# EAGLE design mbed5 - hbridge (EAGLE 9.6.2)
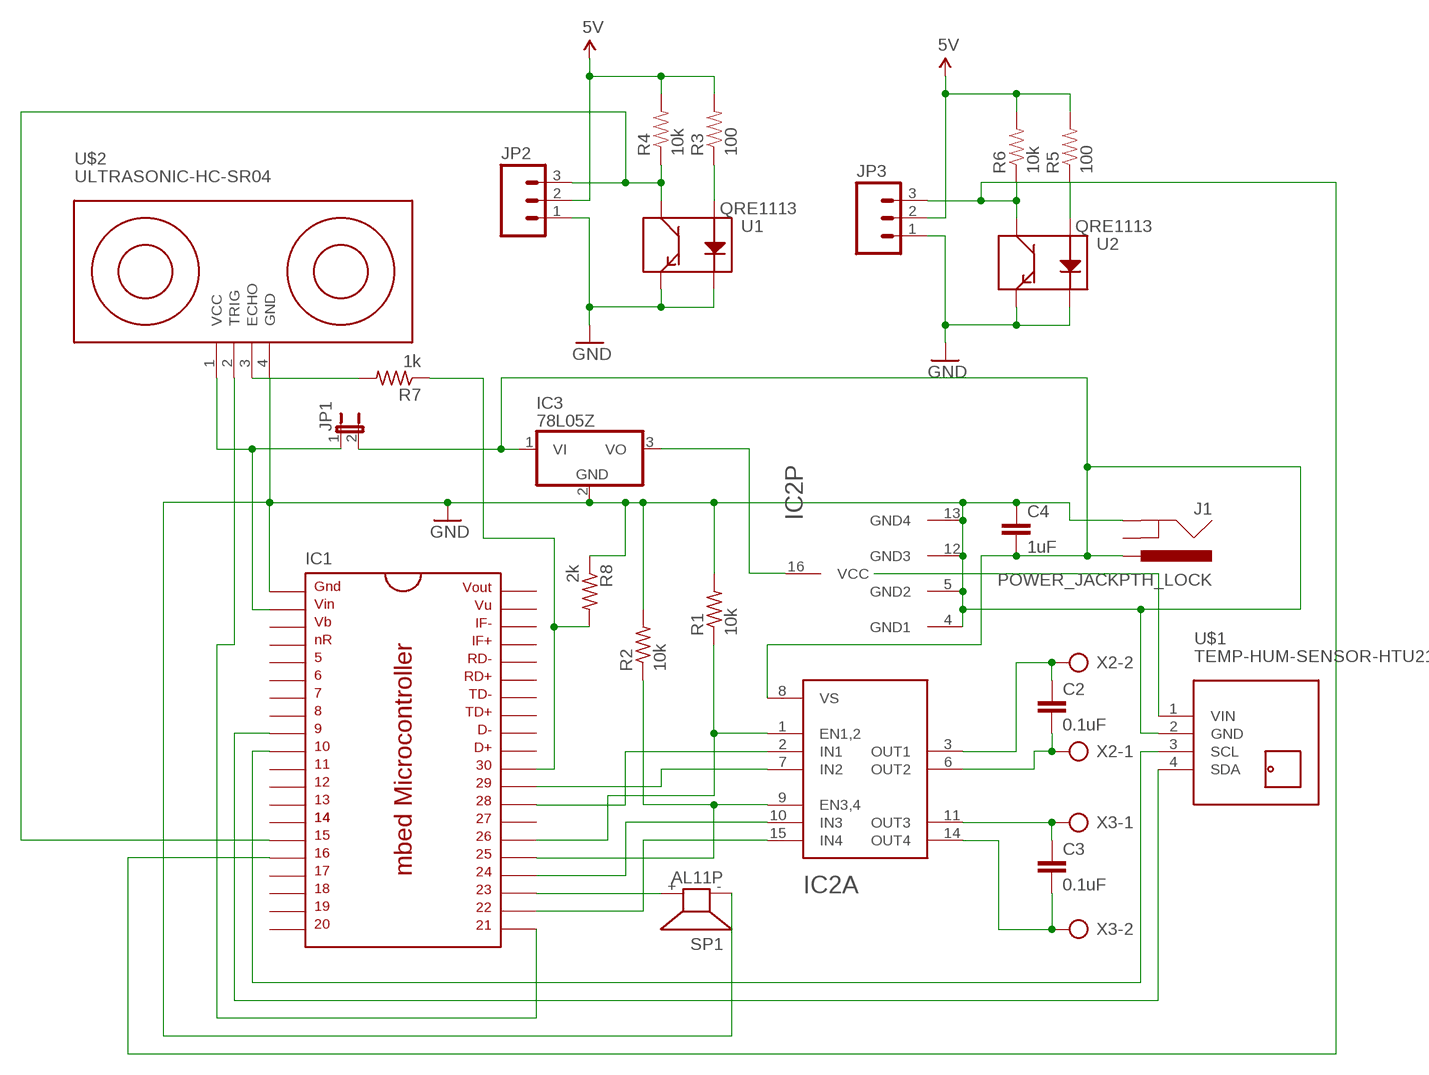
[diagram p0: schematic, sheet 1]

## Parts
C2  0.1uF  C5/3.5  [C5B3.5]
C3  0.1uF  C5/3.5  [C5B3.5]
C4  1uF  C5/3.5  [C5B3.5]
IC1  MBED_MICROCONTROLLER  [DIL40_0.9]
IC2  L293D  [DIP16]
IC3  78L05Z  [TO92]
J1  POWER_JACKPTH_LOCK  [POWER_JACK_PTH_LOCK]
JP1  JUMPER-2PTH  [1X02]
JP2  M03SMD_RA_MALE  [1X03_SMD_RA_MALE]
JP3  M03SMD_RA_MALE  [1X03_SMD_RA_MALE]
R1  10k  R-US_0207/10  [0207/10]
R2  10k  R-US_0207/10  [0207/10]
R3  100  100-1%  [0402-RES]
R4  10k  10KOHM1/10W1%(0603)  [0402-RES]
R5  100  100-1%  [0402-RES]
R6  10k  10KOHM1/10W1%(0603)  [0402-RES]
R7  1k  R-US_0207/10  [0207/10]
R8  2k  R-US_0207/10  [0207/10]
SP1  AL11P  [AL11P]
U1  QRE1113  [QRE1113]
U2  QRE1113  [QRE1113]
U$1  TEMP-HUM-SENSOR-HTU21D  [TEMP-HUM-SENSOR-HTU21D]
U$2  ULTRASONIC-HC-SR04  [ULTRASONIC-HC-SR04]
X2  AK300/2  [AK300/2]
X3  AK300/2  [AK300/2]

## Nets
5V: JP2.2 JP3.2 R3.2 R4.2 R5.2 R6.2
GND: JP2.1 JP3.1 U1.2(K) U1.4(E) U2.2(K) U2.4(E)
N$1: IC1.22 IC2.15(A:IN4)
N$2: IC1.24 IC2.10(A:IN3)
N$3: IC1.25 IC2.9(A:EN3,4) R2.1
N$4: IC1.28 IC2.2(A:IN1)
N$5: IC1.29 IC2.7(A:IN2)
N$6: IC1.26 IC2.1(A:EN1,2) R1.1
N$7: IC1.9 U$1.4(SDA)
N$8: C2.1 IC2.3(A:OUT1) X2.2
N$9: C2.2 IC2.6(A:OUT2) X2.1
N$10: C3.1 IC2.11(A:OUT3) X3.1
N$11: C3.2 IC2.14(A:OUT4) X3.2
N$12: IC2.16(P:VCC) IC3.3(VO)
N$13: IC1.2 JP1.1 U$2.1(VCC)
N$14: C4.1 C4.2 IC1.1 IC2.4(P:GND1) IC2.5(P:GND2) IC2.8(A:VS) IC2.12(P:GND3) IC2.13(P:GND4) IC3.1(VI) IC3.2(GND) J1.GND J1.PWR JP1.2 R1.2 R2.2 R8.1 SP1.- U$1.2(GND) U$2.4(GND) ; supply symbol labelled GND
N$15: IC1.10 U$1.3(SCL)
N$16: IC1.23 SP1.+
N$17: U$1.1(VIN)
N$18: IC1.21 U$2.2(TRIG)
N$20: R3.1 U1.1(A)
N$21: IC1.15 JP2.3 R4.1 U1.3(C)
N$22: R7.2 U$2.3(ECHO)
N$23: R5.1 U2.1(A)
N$24: IC1.16 JP3.3 R6.1 U2.3(C)
N$25: IC1.30 R7.1 R8.2
Unconnected: IC1.3 IC1.4 IC1.5 IC1.6 IC1.7 IC1.8 IC1.11 IC1.12 IC1.13 IC1.14 IC1.17 IC1.18 IC1.19 IC1.20 IC1.27 IC1.31 IC1.32 IC1.33 IC1.34 IC1.35 IC1.36 IC1.37 IC1.38 IC1.39 IC1.40 J1.GNDBREAK

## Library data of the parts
C2-C4 = capacitor-wima:C: CAPACITOR
IC1 = LPC1768RefDesign:MBED_MICROCONTROLLER: mbed Microcontroller, DIP40, 0.9"
IC2 = ads:L293D: L293D Quad Half H-Bridge with integrated diodes
IC3 = gm-regulators:78*: Positive VOLTAGE REGULATOR Source: http://cache.national.com/ds/LM/LM78L05.pdf http://www.fairchildsemi.com/ds/LM/LM7805.pdf
J1 = SparkFun-Connectors:POWER_JACK: Power Jack This is the standard 5.5mm barrel jack for power. The PTH is the most common, proven, reliable, footprint. The Slot footprint only works if the mill layer is transmitted to the PCB fab house so be warned. Mating wall wart : TOL-00298 (and others); PROD_ID: PRT-00119
JP1 = SparkFun-Retired:JUMPER-2: Jumper
JP2 JP3 = SparkFun-Connectors:M03: Header 3 Standard 3-pin 0.1" header. Use with straight break away headers (SKU : PRT-00116), right angle break away headers (PRT-00553), swiss pins (PRT-00743), machine pins (PRT-00117), and female headers (PRT-00115). Molex polarized connector foot print use with SKU : PRT-08232 with associated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; PROD_ID: CONN-10925
R1 R2 R7 R8 = adafruit:R-US_: RESISTOR, American symbol
R3 R5 = SparkFun-Resistors:100-1%: 100-ohm SMT; PROD_ID: RES-07863
R4 R6 = SparkFun-Resistors:10KOHM1/10W1%(0603): RES-00824; PROD_ID: RES-00824
SP1 = buzzer:AL11P: SPEAKER; OC_FARNELL: unknown; OC_NEWARK: unknown
U1 U2 = SparkFun-Sensors:QRE1113: Reflective object sensor; PROD_ID: IC-09357
U$1 = diy-modules:TEMP-HUM-SENSOR-HTU21D: Digital Humidity & Temperature Sensor based on HTU21D device More information about HTU21D device is available here: http://futureeverything.org/wp-content/uploads/2014/05/Humidity-Datasheet.pdf HTU21D Arudino Library is available here: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
U$2 = diy-modules:ULTRASONIC-HC-SR04: Ultrasonic Ranging Module HC-SR04 More details available here: http://randomnerdtutorials.com/complete-guide-for-ultrasonic-sensor-hc-sr04/ Click here to find device on ebay.com
X2 X3 = con-ptr500:AK300/2: CONNECTOR; OC_FARNELL: unknown; OC_NEWARK: unknown

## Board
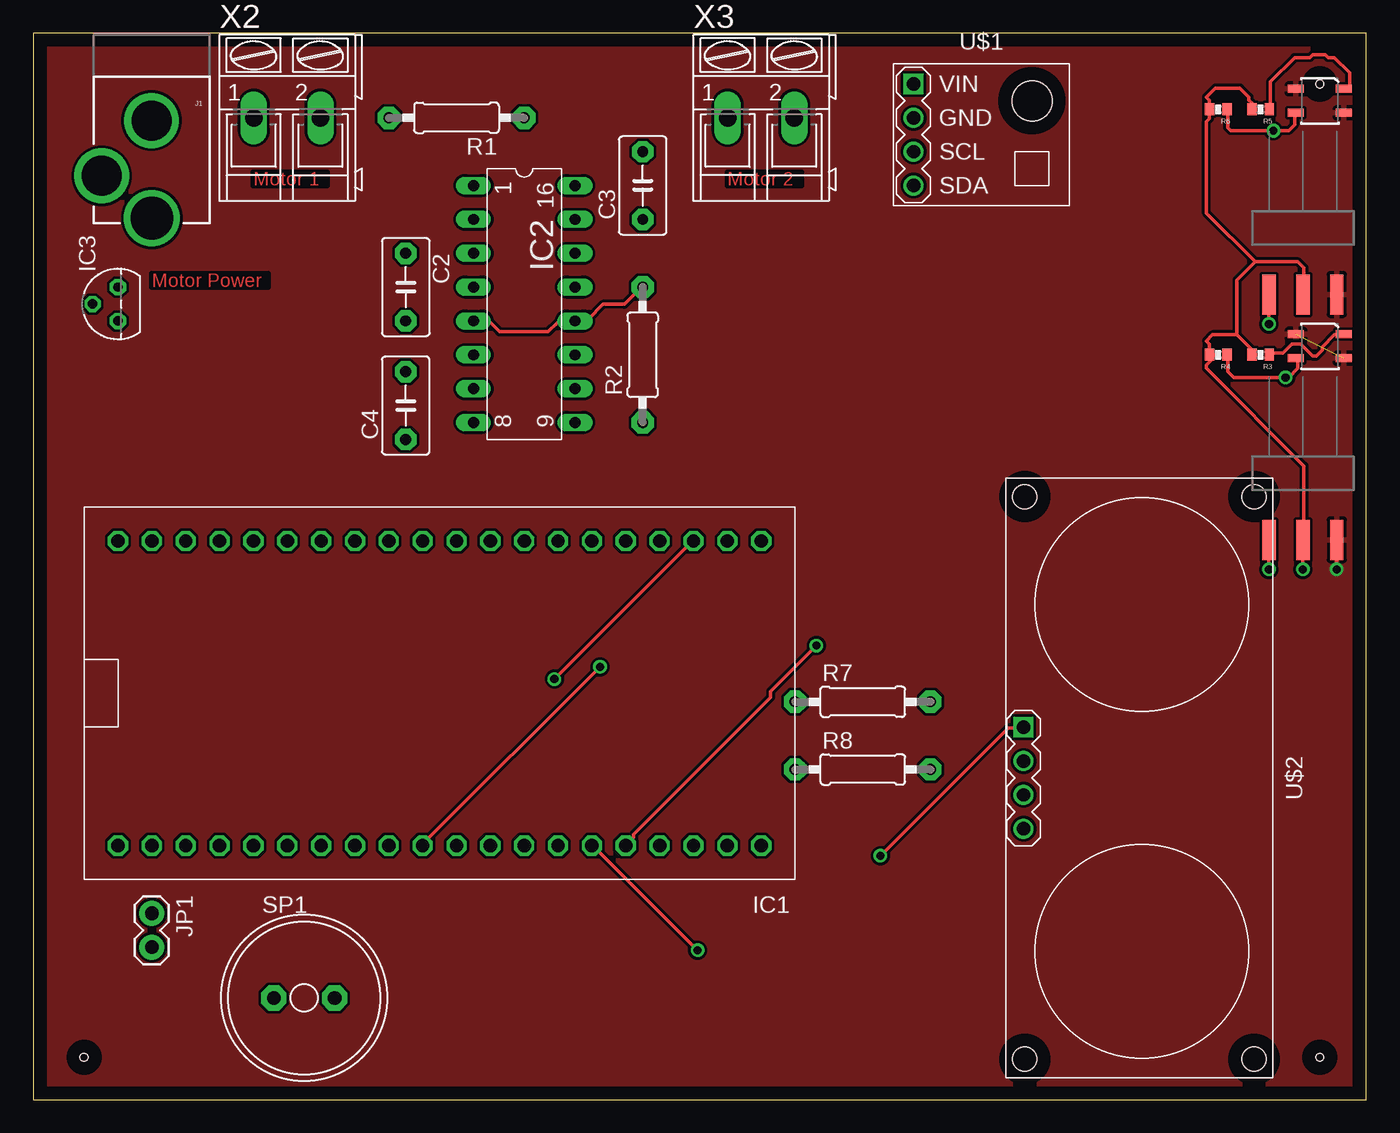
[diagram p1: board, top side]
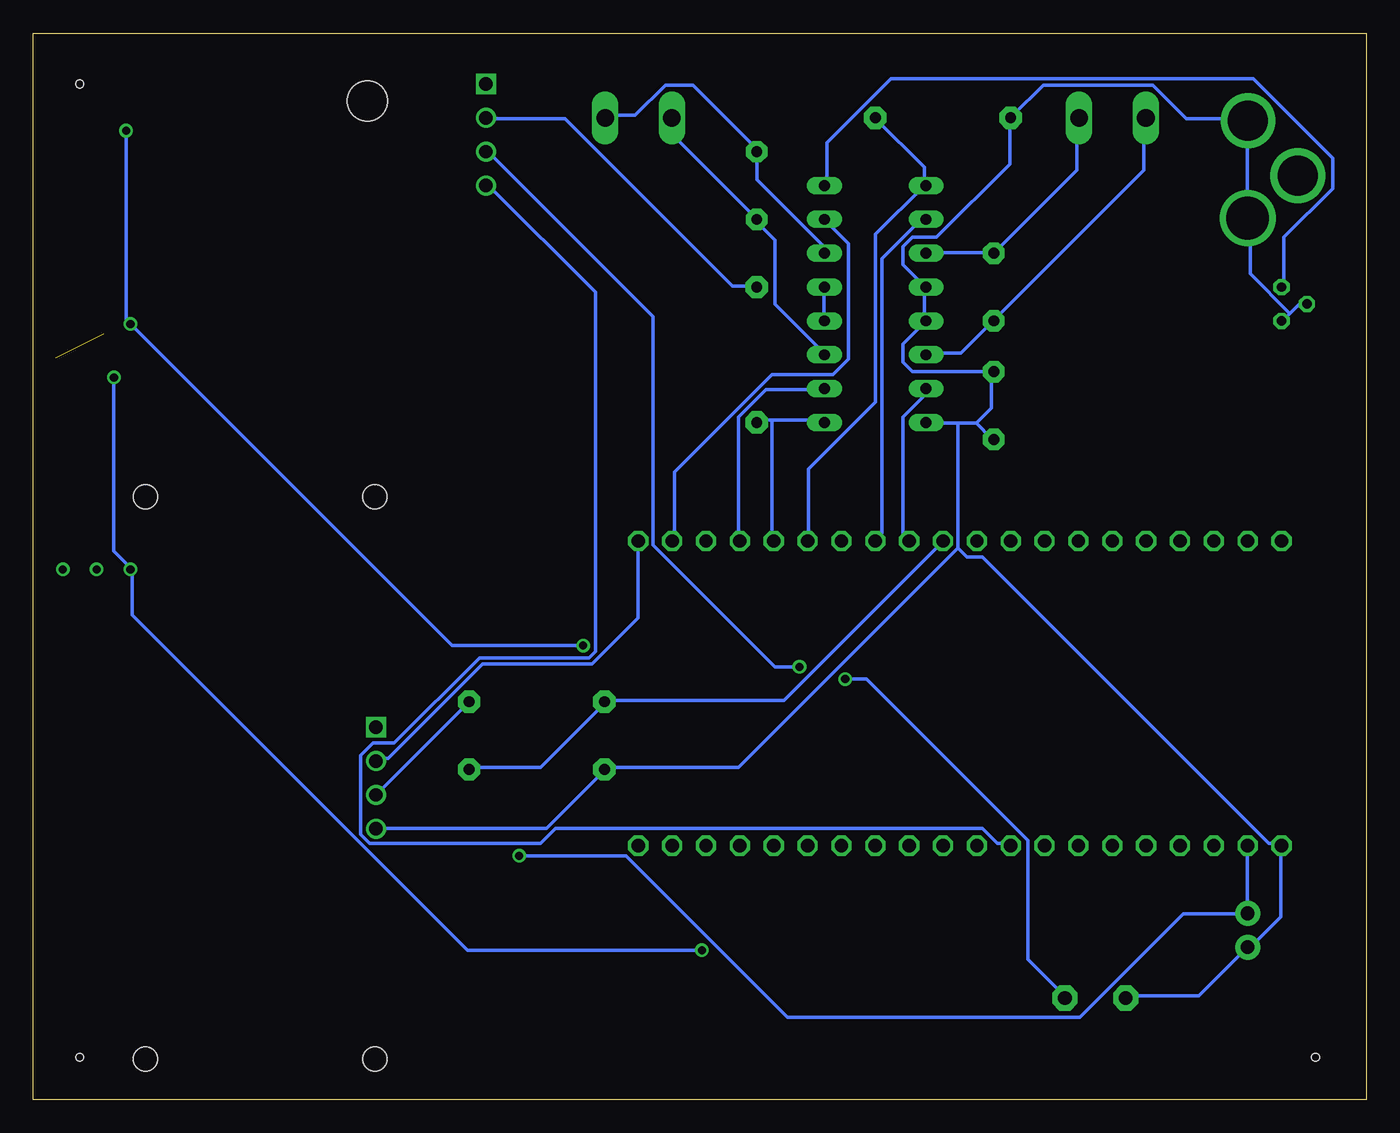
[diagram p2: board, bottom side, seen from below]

Size 100 x 80 mm. Coordinates in mm from the lower left corner, seen from the top.
Outline: 0,0 100,0 100,80 0,80 0,0
Copper layers (1*16): Top 0.035mm / dielectric 1.5mm / Bottom 0.035mm
Design rules "default": minimum track width 10mil, minimum drill 24mil, track to track 8mil, track to pad 8mil, pad to pad 8mil, via to via 8mil, smd to smd 8mil, copper to edge 40mil, drill to drill 8mil, minimum pad ring 10mil, minimum via ring 8mil, stop-mask expansion 4mil, vias tented up to drill 0mil, thermal gap 10mil
Holes 0.6 mm at 3.81,3.17 96.52,3.17 96.52,76.2

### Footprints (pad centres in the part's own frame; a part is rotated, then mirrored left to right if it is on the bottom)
C5B3.5 = drill 0.813 pad 1.6 octagon: 1 -2.54,0; 2 2.54,0
DIL40_0.9 = drill 1 pad 1.397 octagon: 1 -22.86,-11.43; 2 -20.32,-11.43; 3 -17.78,-11.43; 4 -15.24,-11.43; 5 -12.7,-11.43; 6 -10.16,-11.43; 7 -7.62,-11.43; 8 -5.08,-11.43; 9 -2.54,-11.43; 10 0,-11.43; 11 2.54,-11.43; 12 5.08,-11.43; 13 7.62,-11.43; 14 10.16,-11.43; 15 12.7,-11.43; 16 15.24,-11.43; 17 17.78,-11.43; 18 20.32,-11.43; 19 22.86,-11.43; 20 25.4,-11.43; 21 25.4,11.43; 22 22.86,11.43; 23 20.32,11.43; 24 17.78,11.43; 25 15.24,11.43; 26 12.7,11.43; 27 10.16,11.43; 28 7.62,11.43; 29 5.08,11.43; 30 2.54,11.43; 31 0,11.43; 32 -2.54,11.43; 33 -5.08,11.43; 34 -7.62,11.43; 35 -10.16,11.43; 36 -12.7,11.43; 37 -15.24,11.43; 38 -17.78,11.43; 39 -20.32,11.43; 40 -22.86,11.43
DIP16 = drill 0.813 long: 1 -8.89,-3.81; 2 -6.35,-3.81; 3 -3.81,-3.81; 4 -1.27,-3.81; 5 1.27,-3.81; 6 3.81,-3.81; 7 6.35,-3.81; 8 8.89,-3.81; 9 8.89,3.81; 10 6.35,3.81; 11 3.81,3.81; 12 1.27,3.81; 13 -1.27,3.81; 14 -3.81,3.81; 15 -6.35,3.81; 16 -8.89,3.81
TO92 = drill 0.7 octagon: 1 -1.27,0; 2 0,1.905; 3 1.27,0
POWER_JACK_PTH_LOCK = drill 2.997 pad 4.115: GND 0.025,6.557; GNDBREAK 3.762,10.7 | drill 3.2 pad 4.115: PWR 0,13.878
1X02 = drill 1.016 pad 1.88: 1 0,0; 2 2.54,0
1X03_SMD_RA_MALE = smd 1 x 3: 1 -2.54,5; 2 0,5; 3 2.54,5
0207/10 = drill 0.813 pad 1.676 octagon: 1 -5.08,0; 2 5.08,0
0402-RES = smd 0.7 x 0.9: 1 -0.65,0; 2 0.65,0
AL11P = drill 1.016 pad 1.905 octagon: + 2.286,0; - -2.286,0
QRE1113 = smd 1.2 x 0.6: 1 -1.8,-0.9; 2 1.8,-0.9; 3 1.8,0.9; 4 -1.8,0.9
TEMP-HUM-SENSOR-HTU21D = drill 1 square: 1 -5.08,3.81 | drill 1: 2 -5.08,1.27; 3 -5.08,-1.27; 4 -5.08,-3.81 | hole 3: 3.81,2.54
ULTRASONIC-HC-SR04 = drill 1 square: 1 -3.81,-8.89 | drill 1: 2 -1.27,-8.89; 3 1.27,-8.89; 4 3.81,-8.89 | hole 1.8: -21.1,8.4; -21.1,-8.8; 21.1,-8.8; 21.1,8.4
AK300/2 = drill 1.321 long: 1 -2.515,0; 2 2.489,0

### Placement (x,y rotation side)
C2  27.94,60.96 270 top
C3  45.72,68.58 90 top
C4  27.94,52.07 90 top
IC1  29.21,30.48 0 top
IC2  36.83,59.69 270 top
IC3  6.35,59.69 90 top
J1  8.89,80.01 180 top
JP1  8.89,13.97 270 top
JP2  95.25,46.99 180 top
JP3  95.25,65.41 180 top
R1  31.75,73.66 180 top
R2  45.72,55.88 90 top
R3  92.08,55.88 180 top
R4  88.9,55.88 180 top
R5  92.08,74.3 180 top
R6  88.9,74.3 180 top
R7  62.23,29.84 0 top
R8  62.23,24.77 0 top
SP1  20.32,7.62 0 top
U1  96.52,56.52 180 top
U2  96.52,74.93 180 top
U$1  71.12,72.39 0 top
U$2  83.19,24.13 270 top
X2  19.05,73.66 0 top
X3  54.61,73.66 0 top

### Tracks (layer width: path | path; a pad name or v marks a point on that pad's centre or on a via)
5V  (via drill 0.61)
  Top 0.254: v95.25,39.78 JP2.2 95.33,42.06 95.33,47.55 88.01,54.86 88.01,55.09 88.7,55.78 88.47,56.01 R4.2 88.24,56.01 88.24,56.69 88.01,56.92 88.47,57.38 90.3,57.38 | R6.2 88.24,74.98 88.01,75.21 88.7,75.89 90.53,75.89 91.21,75.21 91.21,74.98 91.44,74.75 91.44,74.3 R5.2 | 90.3,57.38 91.67,56.01 91.44,55.78 R3.2 | 90.3,57.38 90.3,61.49 91.67,62.87 | 91.67,62.87 94.87,62.87 95.33,62.41 95.33,60.58 JP3.2 | R6.2 88.24,73.61 88.01,73.38 88.01,66.52 91.67,62.87 | R6.2
GND  (via drill 0.61)  (1 unrouted)
  Top 0.254: JP2.1 v97.79,39.78
  pour Top: 0,80.01 0,0 100.33,0 100.33,80.01
N$1
  Bottom 0.254: IC2.15 40.46,65.84 38.86,64.24 38.86,55.55 40.01,54.41 44.58,54.41 51.89,47.09 51.89,42.06 IC1.22
N$2
  Bottom 0.254: IC2.10 40.69,53.26 45.03,53.26 47.09,51.21 47.09,42.06 IC1.24
N$3
  Bottom 0.254: 44.58,50.98 45.72,50.98 R2.1 | 44.58,50.98 40.69,50.98 IC2.9 | 44.58,50.98 44.58,42.06 IC1.25
N$4
  Bottom 0.254: IC2.2 33.15,65.84 33.6,65.84 36.35,63.09 36.35,42.52 36.8,42.06 IC1.28
N$5
  Bottom 0.254: IC2.7 33.15,53.26 33.15,52.81 34.75,51.21 34.75,42.52 34.29,42.06 IC1.29
N$6
  Bottom 0.254: 33.15,68.58 33.15,69.95 36.8,73.61 R1.1 | 33.15,68.58 36.8,64.92 36.8,52.35 41.83,47.32 41.83,42.06 IC1.26 | 33.15,68.58 IC2.1
N$7
  Bottom 0.254: IC1.9 26.75,19.2 27.66,19.2 28.8,20.34 60.81,20.34 61.95,19.2 74.75,19.2 75.44,19.89 75.44,25.83 74.52,26.75 72.92,26.75 66.52,33.15 58.29,33.15 57.84,33.6 57.84,60.58 65.84,68.58 U$1.4
N$8
  Bottom 0.254: IC2.3 32.92,63.55 28.12,63.55 C2.1 21.72,69.72 21.72,73.61 X2.2
N$9
  Bottom 0.254: IC2.6 32.92,56.01 30.4,56.01 28.12,58.29 C2.2 27.89,58.52 16.69,69.72 16.69,73.61 X2.1
N$10
  Bottom 0.254: IC2.11 40.69,56.01 44.35,59.66 44.35,64.47 45.72,65.84 C3.1 45.72,66.06 51.89,72.24 51.89,73.61 X3.1
N$11
  Bottom 0.254: IC2.14 40.69,63.55 40.69,64.01 45.72,69.04 C3.2 45.72,71.32 50.52,76.12 52.58,76.12 54.86,73.84 56.92,73.84 X3.2
N$12
  Bottom 0.254: IC3.3 6.17,61.04 6.17,64.69 2.52,68.35 2.52,70.64 8.46,76.58 35.66,76.58 40.46,71.78 40.46,68.58 IC2.16
N$13  (via drill 0.61)
  Top 0.254: v63.55,18.29 73.15,27.89 74.3,27.89 U$2.1
  Bottom 0.254: IC1.2 8.91,18.97 8.91,14.17 JP1.1 8.91,13.95 13.72,13.95 21.49,6.17 43.43,6.17 55.55,18.29 v63.55,18.29
N$14
  Top 0.254: R2.2 45.72,61.04 44.35,59.66 42.75,59.66 41.6,58.52 40.69,58.52 IC2.12 40.46,58.29 39.32,58.29 38.63,57.61 34.98,57.61 34.29,58.29 33.15,58.29 IC2.5
  Bottom 0.254: IC2.12 40.69,58.52 40.69,60.81 IC2.13 | U$1.2 65.84,73.61 60.12,73.61 47.55,61.04 45.72,61.04 R2.2 | 5.71,58.98 6.17,58.52 IC3.1 | 5.71,58.98 5.03,59.66 4.57,59.66 IC3.2 | 5.71,58.98 8.69,61.95 8.69,66.06 J1.PWR 8.91,66.29 8.91,73.38 J1.GND 8.91,73.61 13.49,73.61 16,76.12 24.23,76.12 26.52,73.84 R1.2 26.75,73.61 26.75,70.18 32.23,64.69 34.06,64.69 34.75,64.01 34.75,62.64 33.15,61.04 IC2.4 33.15,60.81 33.15,58.52 IC2.5 34.75,56.69 34.75,55.32 34.06,54.63 28.12,54.63 C4.2 28.12,54.41 28.12,51.89 29.26,50.75 | SP1.- 17.83,7.77 12.57,7.77 8.91,11.43 JP1.2 8.69,11.43 6.4,13.72 6.4,18.97 IC1.1 6.4,19.2 7.32,19.2 28.8,40.69 29.95,40.69 30.63,41.38 | U$2.4 74.3,20.34 61.49,20.34 57.15,24.69 R8.1 57.15,24.92 47.09,24.92 30.63,41.38 | 29.26,50.75 30.63,50.75 | 30.63,50.75 32.92,50.75 IC2.8 | 29.26,50.75 28.12,49.61 C4.1 | 30.63,50.75 30.63,41.38
N$15  (via drill 0.61)
  Top 0.254: v42.52,32.46 29.26,19.2 IC1.10
  Bottom 0.254: v42.52,32.46 44.35,32.46 53.49,41.6 53.49,58.75 65.84,71.09 U$1.3
N$16  (via drill 0.61)
  Top 0.254: v39.09,31.55 49.38,41.83 IC1.23
  Bottom 0.254: v39.09,31.55 37.49,31.55 25.38,19.43 25.38,10.52 22.63,7.77 SP1.+
N$18
  Bottom 0.254: U$2.2 74.3,25.6 73.38,25.6 66.29,32.69 58.06,32.69 54.63,36.12 54.63,41.83 IC1.21
N$20
  Top 0.254: R3.1 92.81,56.01 93.73,56.01 94.41,56.69 95.1,56.69 96.01,55.78 96.24,55.78 96.7,56.24 96.7,56.46 97.61,57.38 98.3,57.38 U1.1
N$21  (via drill 0.61)
  Top 0.254: JP2.3 v92.71,39.78 | R4.1 89.61,55.78 89.61,54.63 90.07,54.18 v93.95,54.18 94.18,54.18 94.87,54.86 94.87,55.55 U1.3 | v49.84,11.2 42.06,18.97 IC1.15
  Bottom 0.254: v49.84,11.2 67.44,11.2 92.58,36.35 92.58,39.78 v92.71,39.78 92.81,40.01 93.95,41.15 v93.95,54.18
N$22
  Bottom 0.254: R7.2 U$2.3
N$23
  Top 0.254: R5.1 92.81,74.3 92.81,76.35 94.64,78.18 95.78,78.18 96.01,78.41 96.93,78.41 97.16,78.18 97.61,78.18 98.75,77.04 98.75,75.89 98.53,75.67 U2.1
N$24  (via drill 0.61)
  Top 0.254: JP3.3 v92.71,58.19 | R6.1 89.61,74.3 89.61,72.92 89.84,72.69 v93.04,72.69 94.18,72.69 94.64,73.15 94.64,73.84 U2.3 | v58.75,34.06 55.32,30.63 55.32,30.18 45.03,19.89 45.03,19.66 44.58,19.2 IC1.16
  Bottom 0.254: v58.75,34.06 68.58,34.06 92.58,58.06 v92.71,58.19 92.81,58.29 93.04,58.52 v93.04,72.69
N$25
  Bottom 0.254: IC1.30 31.77,41.83 43.66,29.95 57.15,29.95 R7.1 57.15,29.72 61.95,24.92 67.21,24.92 R8.2

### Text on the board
Top: Motor 1 | Motor 2 | Motor Power

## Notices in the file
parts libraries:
SparkFun-Connectors: Licensing: Creative Commons ShareAlike 4.0 International - https://creativecommons.org/licenses/by-sa/4.0
diy-modules: Released under the Creative Commons Attribution 4.0 International License: http://creativecommons.org/licenses/by/4.0
